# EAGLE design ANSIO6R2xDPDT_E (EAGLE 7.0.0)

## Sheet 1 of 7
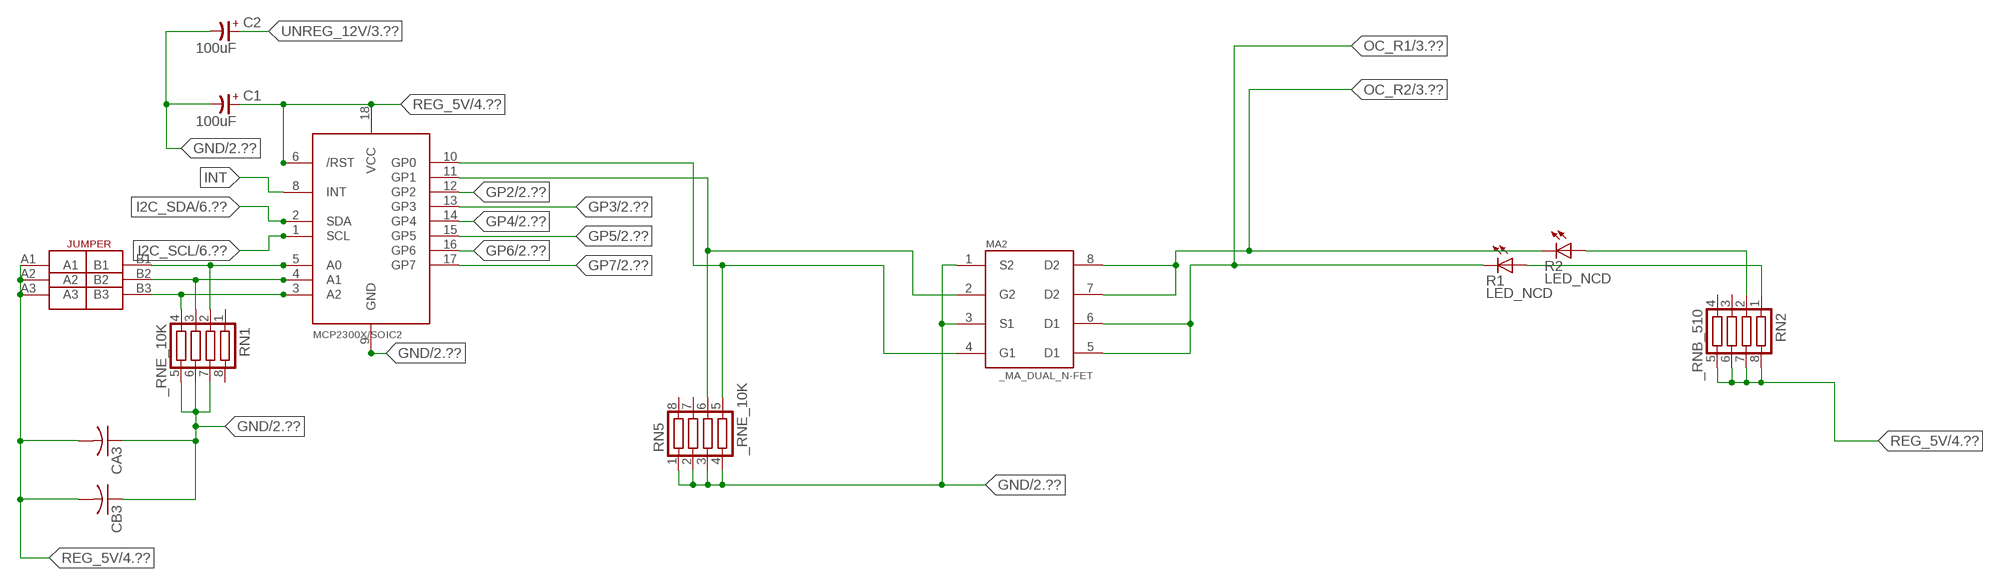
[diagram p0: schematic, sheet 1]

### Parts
C1  100uF  CP-E-025X060  [E-025X060]
C2  100uF  CP-E-025X060  [E-025X060]
CA3  CC1206KRX7R9BB104C1206K  [CC1206KRX7R9BB104]
CB3  TMK316F106ZL-TC1206K  [TMK316F106ZL-T]
IC2  MCP2300X/SO  [SO18W]
MA2  _MA_DUAL_N-FET  [_MA_DUAL_N-FET]
R1  LED_NCD  [CHIPLED_0603]
R2  LED_NCD  [CHIPLED_0603]
RN1  _RNE_10K  [RNE]
RN2  _RNB_510  [RNB]
RN5  _RNE_10K  [RNE]
U$18  JUMPER_3X2  [JUMPER_3X2]

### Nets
GND: C1.- C2.- CA3.1 CB3.1 IC2.9(GND) MA2.1(S2) MA2.3(S1) RN1.5 RN1.6 RN1.7 RN5.1 RN5.2 RN5.3 RN5.4 ; also sheet 2,4,5,6,7
GP2: IC2.12(GP2) ; also sheet 2
GP3: IC2.13(GP3) ; also sheet 2
GP4: IC2.14(GP4) ; also sheet 2
GP5: IC2.15(GP5) ; also sheet 2
GP6: IC2.16(GP6) ; also sheet 2
GP7: IC2.17(GP7) ; also sheet 2
I2C_SCL: IC2.1(SCL) ; also sheet 6,7
I2C_SDA: IC2.2(SDA) ; also sheet 6,7
INT: IC2.8(INT)
N$6: IC2.5(A0) RN1.2 U$18.B1
N$7: IC2.4(A1) RN1.3 U$18.B2
N$8: IC2.3(A2) RN1.4 U$18.B3
N$22: IC2.11(GP1) MA2.2(G2) RN5.6
N$23: IC2.10(GP0) MA2.4(G1) RN5.5
N$31: R2.A RN2.2
N$32: R1.A RN2.1
OC_R1: MA2.5(D1) MA2.6(D1) R1.C ; also sheet 3
OC_R2: MA2.7(D2) MA2.8(D2) R2.C ; also sheet 3
REG_5V: C1.+ CA3.2 CB3.2 IC2.6(/RST) IC2.18(VCC) RN2.5 RN2.6 RN2.7 RN2.8 U$18.A1 U$18.A2 U$18.A3 ; also sheet 4,5,6,7
UNREG_12V: C2.+ ; also sheet 3,4
Unconnected: RN1.1 RN1.8 RN2.3 RN2.4 RN5.7 RN5.8

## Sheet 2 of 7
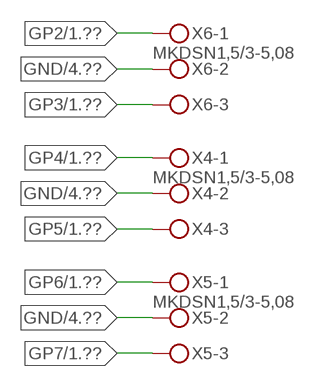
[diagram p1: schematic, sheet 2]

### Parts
X4  MKDSN1,5/3-5,08  [MKDSN1,5/3-5,08]
X5  MKDSN1,5/3-5,08  [MKDSN1,5/3-5,08]
X6  MKDSN1,5/3-5,08  [MKDSN1,5/3-5,08]

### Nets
GND: X4.2 X5.2 X6.2 ; also sheet 1,4,5,6,7
GP2: X6.1 ; also sheet 1
GP3: X6.3 ; also sheet 1
GP4: X4.1 ; also sheet 1
GP5: X4.3 ; also sheet 1
GP6: X5.1 ; also sheet 1
GP7: X5.3 ; also sheet 1

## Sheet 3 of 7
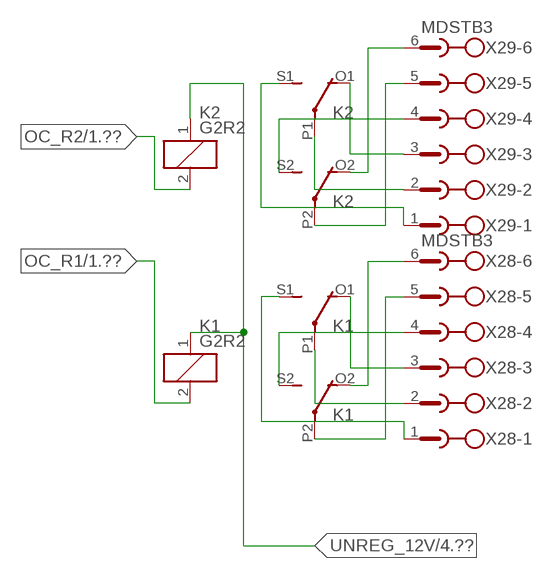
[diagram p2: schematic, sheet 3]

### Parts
K1  G2R2  [G2R2]
K2  G2R2  [G2R2]
X28  MDSTB3  [MDSTB3]
X29  MDSTB3  [MDSTB3]

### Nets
N$203: K1.P2(3:COM) X28.5
N$204: K1.O2(3:NC) X28.6
N$205: K1.S2(3:NO) X28.4
N$206: K1.P1(2:COM) X28.2
N$207: K1.O1(2:NC) X28.3
N$208: K1.S1(2:NO) X28.1
N$209: K2.P2(3:COM) X29.5
N$210: K2.O2(3:NC) X29.6
N$211: K2.S2(3:NO) X29.4
N$212: K2.S1(2:NO) X29.1
N$213: K2.P1(2:COM) X29.2
N$214: K2.O1(2:NC) X29.3
OC_R1: K1.2(1:C2) ; also sheet 1
OC_R2: K2.2(1:C2) ; also sheet 1
UNREG_12V: K1.1(1:C1) K2.1(1:C1) ; also sheet 1,4

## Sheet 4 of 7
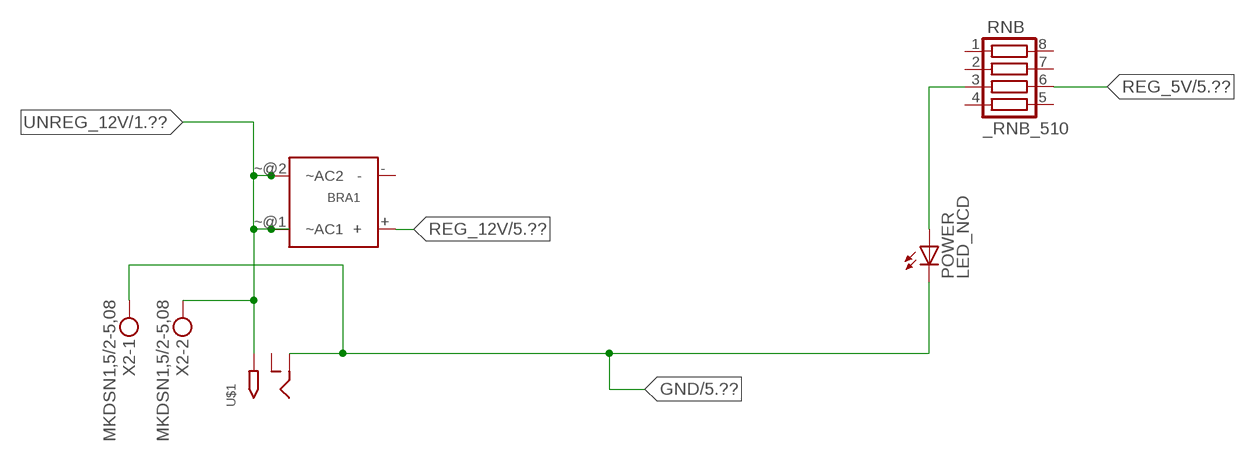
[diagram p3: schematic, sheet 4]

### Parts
BRA1  MB2S_  [MB2S]
POWER  LED_NCD  [CHIPLED_0603]
RNB  _RNB_510  [RNB]
U$1  2.1MMJACK  [PJ-102A]
X2  MKDSN1,5/2-5,08  [MKDSN1,5/2-5,08]

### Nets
GND: POWER.C U$1.RING X2.1 ; also sheet 1,2,5,6,7
N$2: POWER.A RNB.3
REG_5V: RNB.6 ; also sheet 1,5,6,7
REG_12V: BRA1.+ ; also sheet 5
UNREG_12V: BRA1.~@1(~AC1) BRA1.~@2(~AC2) U$1.TIP X2.2 ; also sheet 1,3
Unconnected: BRA1.- RNB.1 RNB.2 RNB.4 RNB.5 RNB.7 RNB.8 U$1.RING_SW

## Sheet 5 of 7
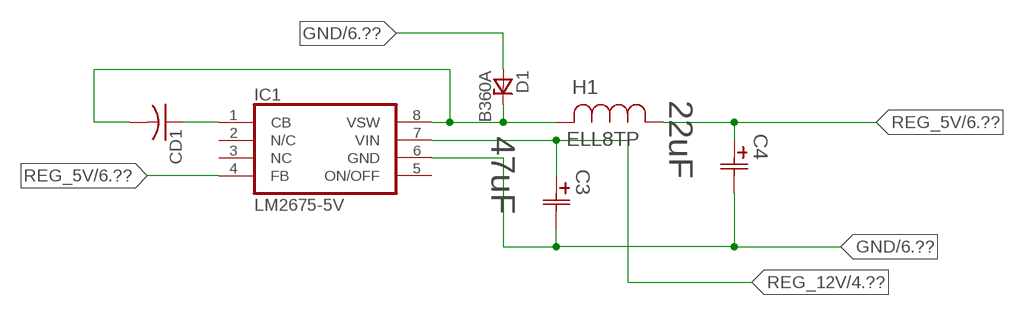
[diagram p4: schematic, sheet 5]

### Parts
C3  47uF  490-5463-6-NDCAP  [C2917(7343)-Y]
C4  22uF  490-5463-6-NDCAP  [C2917(7343)-Y]
CD1  _CD_10NF_50VC1206K  [_CD_10NF_50V]
D1  B360A  [DO214AC_ZENER]
H1  ELL8TP  [IND_ELL8TP]
IC1  LM2675-5V  LM2675  [SO-8]

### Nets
GND: C3.2(C2) C4.2(C2) D1.A IC1.6(GND) ; also sheet 1,2,4,6,7
N$1: CD1.2 D1.C H1.2 IC1.8(VSW)
N$3: CD1.1 IC1.1(CB)
REG_5V: C4.1(C1) H1.1 IC1.4(FB) ; also sheet 1,4,6,7
REG_12V: C3.1(C1) IC1.7(VIN) ; also sheet 4
Unconnected: IC1.2(N/C) IC1.5(ON/OFF)

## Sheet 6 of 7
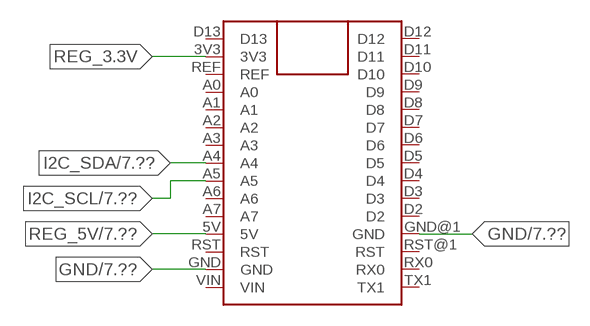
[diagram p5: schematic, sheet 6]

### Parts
FOR_NANO  ARDUINO_NANO  [ARDUINO_NANO]

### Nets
GND: FOR_NANO.GND FOR_NANO.GND@1(GND) ; also sheet 1,2,4,5,7
I2C_SCL: FOR_NANO.A5 ; also sheet 1,7
I2C_SDA: FOR_NANO.A4 ; also sheet 1,7
REG_3.3V: FOR_NANO.3V3
REG_5V: FOR_NANO.5V ; also sheet 1,4,5,7
Unconnected: FOR_NANO.A0 FOR_NANO.A1 FOR_NANO.A2 FOR_NANO.A3 FOR_NANO.A6 FOR_NANO.A7 FOR_NANO.D2 FOR_NANO.D3 FOR_NANO.D4 FOR_NANO.D5 FOR_NANO.D6 FOR_NANO.D7 FOR_NANO.D8 FOR_NANO.D9 FOR_NANO.D10 FOR_NANO.D11 FOR_NANO.D12 FOR_NANO.D13 FOR_NANO.REF FOR_NANO.RST FOR_NANO.RST@1(RST) FOR_NANO.RX0 FOR_NANO.TX1 FOR_NANO.VIN

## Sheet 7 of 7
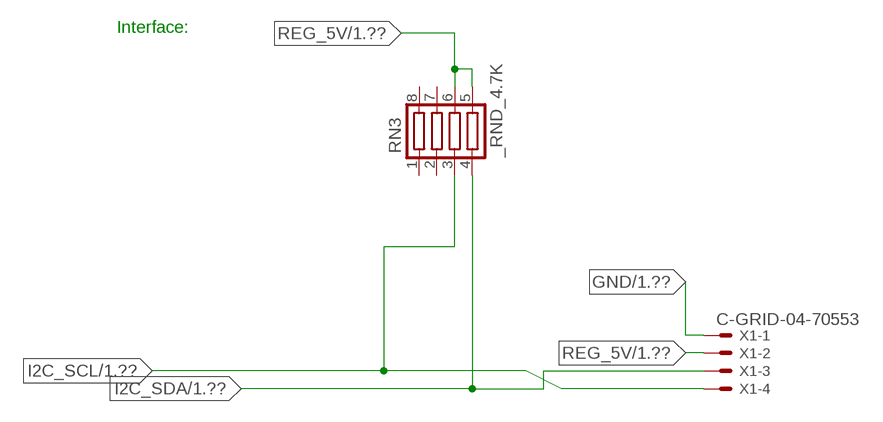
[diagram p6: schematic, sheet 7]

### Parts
RN3  _RND_4.7K  [RND]
X1  C-GRID-04-70553  [70553-04]

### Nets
GND: X1.1 ; also sheet 1,2,4,5,6
I2C_SCL: RN3.3 X1.4 ; also sheet 1,6
I2C_SDA: RN3.4 X1.3 ; also sheet 1,6
REG_5V: RN3.5 RN3.6 X1.2 ; also sheet 1,4,5,6
Unconnected: RN3.1 RN3.2 RN3.7 RN3.8

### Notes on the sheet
- Interface:

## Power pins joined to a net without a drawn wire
NC: IC1.3(NC)

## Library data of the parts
BRA1 = NCD_ULTIMATE_LIBRARY:MB2S: Bridge Rectifier BRA MB2S 200V 500ma Digikey MB2S-TPMSTR-ND/MB2S-TP
C1 C2 = NCD_ULTIMATE_LIBRARY:CP-: Capacitors All Kinds POLARIZED CAP
C3 C4 = NCD_ULTIMATE_bhaskar:490-5463-6-ND: NCD CAP
CA3 = NCD_ULTIMATE_LIBRARY:CC1206KRX7R9BB104: Capacitor CA .1uF 50V SMT C1206K CC1206KRX7R9BB104
CB3 = NCD_ULTIMATE_LIBRARY:TMK316F106ZL-T: Capacitor CB 10uF SMT 1206 TMK316F106ZL-T
CD1 = NCD_ULTIMATE_LIBRARY:_CD_10NF_50V: Capacitor 10nF SMT
D1 = NCD_ULTIMATE_bhaskar:B360A: NCD DIODE B350A/B360A
FOR_NANO = NCD_ULTIMATE_CONNECTORS:ARDUINO_NANO
H1 = NCD_ULTIMATE_bhaskar:ELL8TP: NCD coil
IC1 = NCD_ULTIMATE_bhaskar:LM2675: LM2675 NCD http://www.ti.com/lit/ds/symlink/lm2675.pdf
IC2 = NCD_ULTIMATE_LIBRARY:MCP2300X: Semiconductor Port Expander I/O 8-Bit I2C MCP23008 Inexpensive i2c i/o expander - 8 general purpose i/o pins with optional pullups
K1 K2 = NCD_ULTIMATE_LIBRARY:G2R2: RELAY 2 x switch, Omron
MA2 = NCD_ULTIMATE_LIBRARY:_MA_DUAL_N-FET: FET Dual N-Channel 8-SOIC NMOSFET Digikey 785-1064-2-ND/AO4842
POWER = NCD_ULTIMATE_bhaskar:LED_NCD
R1 R2 = NCD_ULTIMATE_LIBRARY:LED_NCD: LED Digikey 754-1132-2-ND/APT2012SRCPRV
RN1 RN5 = NCD_ULTIMATE_LIBRARY:_RNE_10K: Resistor Array RNE SMT 10K x 4 Single Resistor Source: http://www.ctscorp.com/components/Datasheets/CTSChipArrayDs.pdf Digikey 742C083103JPTR-ND/742C083103JP; OC_FARNELL: unknown; OC_NEWARK: unknown
RN2 RNB = NCD_ULTIMATE_LIBRARY:_RNB_510: Resistor Array RNB SMT 510 x 4 Single Resistor Source: http://www.ctscorp.com/components/Datasheets/CTSChipArrayDs.pdf Digikey 742C083511JPTR-ND/ 742C083511JP; OC_FARNELL: unknown; OC_NEWARK: unknown
RN3 = NCD_ULTIMATE_LIBRARY:_RND_4.7K: Resistor Array RND SMT 4.7K x 4 Single Resistor Source: http://www.ctscorp.com/components/Datasheets/CTSChipArrayDs.pdf Digikey 742C083472JPTR-ND/742C083472JP; OC_FARNELL: unknown; OC_NEWARK: unknown
U$1 = NCD_ULTIMATE_CONNECTORS:2.1MMJACK: 2.1mm x 5.5mm DC jack with internal switch. Digikey part #PJ-102A, 4UCON part #05537 By microbuilder.eu
U$18 = NCD_ULTIMATE_CONNECTORS:JUMPER_3X2
X1 = NCD_ULTIMATE_CONNECTORS:C-GRID-04: CONNECTOR 4-Pos I2C wire to board 2.54 mm (0.100") pitch header Digikey WM1342-ND/0015912045; OC_FARNELL: unknown; OC_NEWARK: unknown
X2 = NCD_ULTIMATE_CONNECTORS:MKDSN1,5/2-5,08: MKDSN 1,5/ 2-5,08 Printklemme
X4-X6 = NCD_ULTIMATE_CONNECTORS:MKDSN1,5/3-5,08: MKDSN 1,5/ 3-5,08 Printklemme Nennstrom: 13,5 A Nennspannung: 250 V Rastermaß: 5,08 mm Polzahl: 3 Anschlussart: Schraubanschluss Montage: Löten Anschlussrichtung Leiter/Platine: 0 ° Artikelnummer: 1729131 Source: http://eshop.phoenixcontact.com .. 1729131.pdf
X28 X29 = NCD_ULTIMATE_LIBRARY:MDSTB3: PHOENIX

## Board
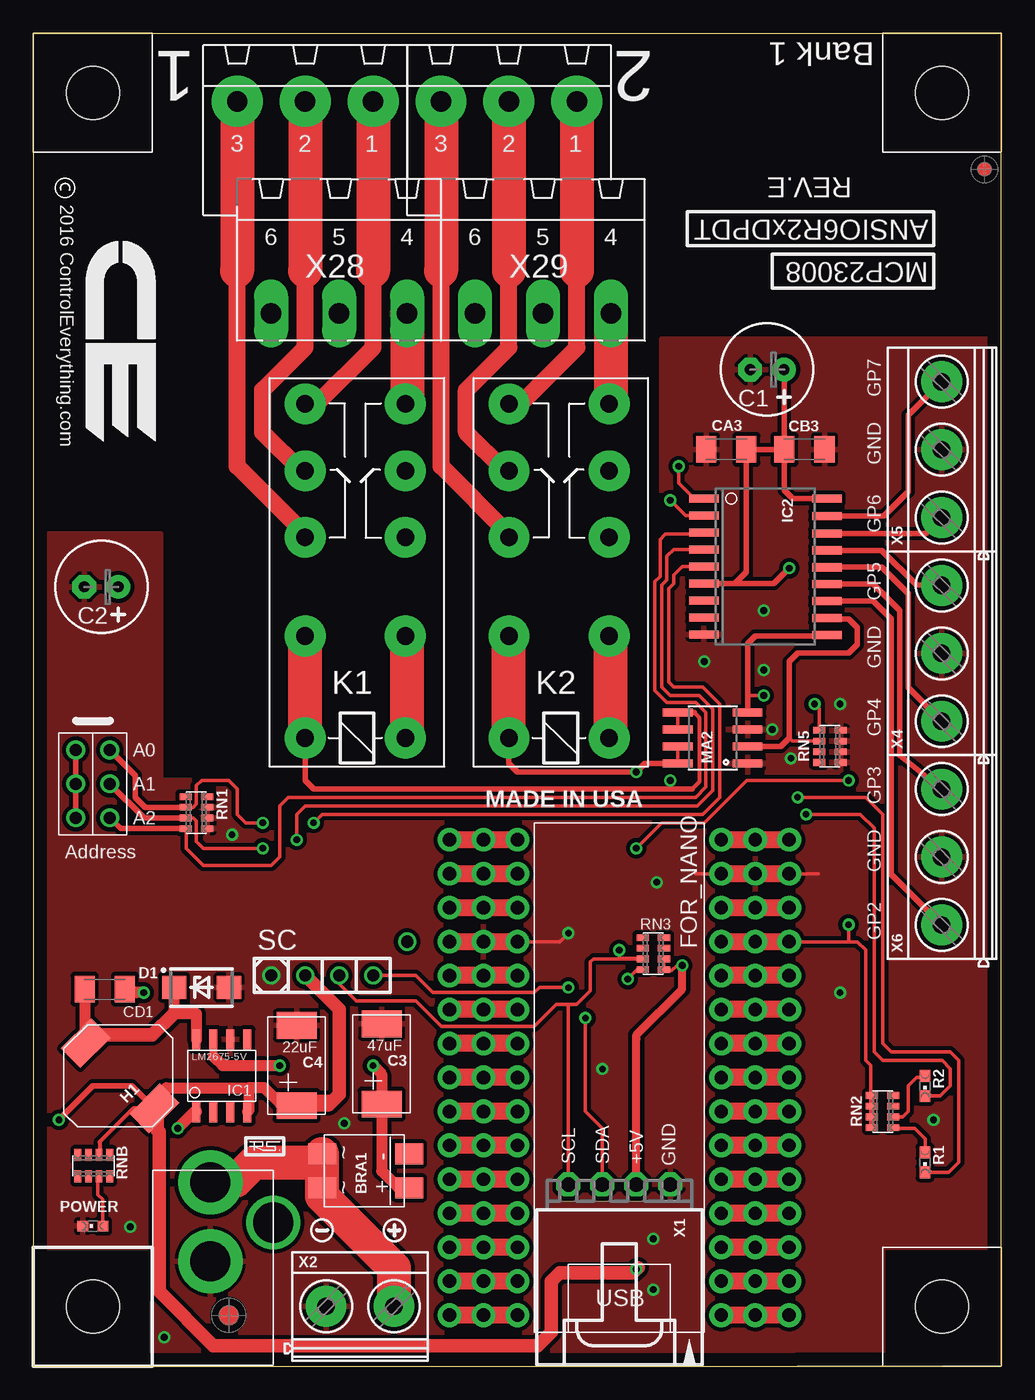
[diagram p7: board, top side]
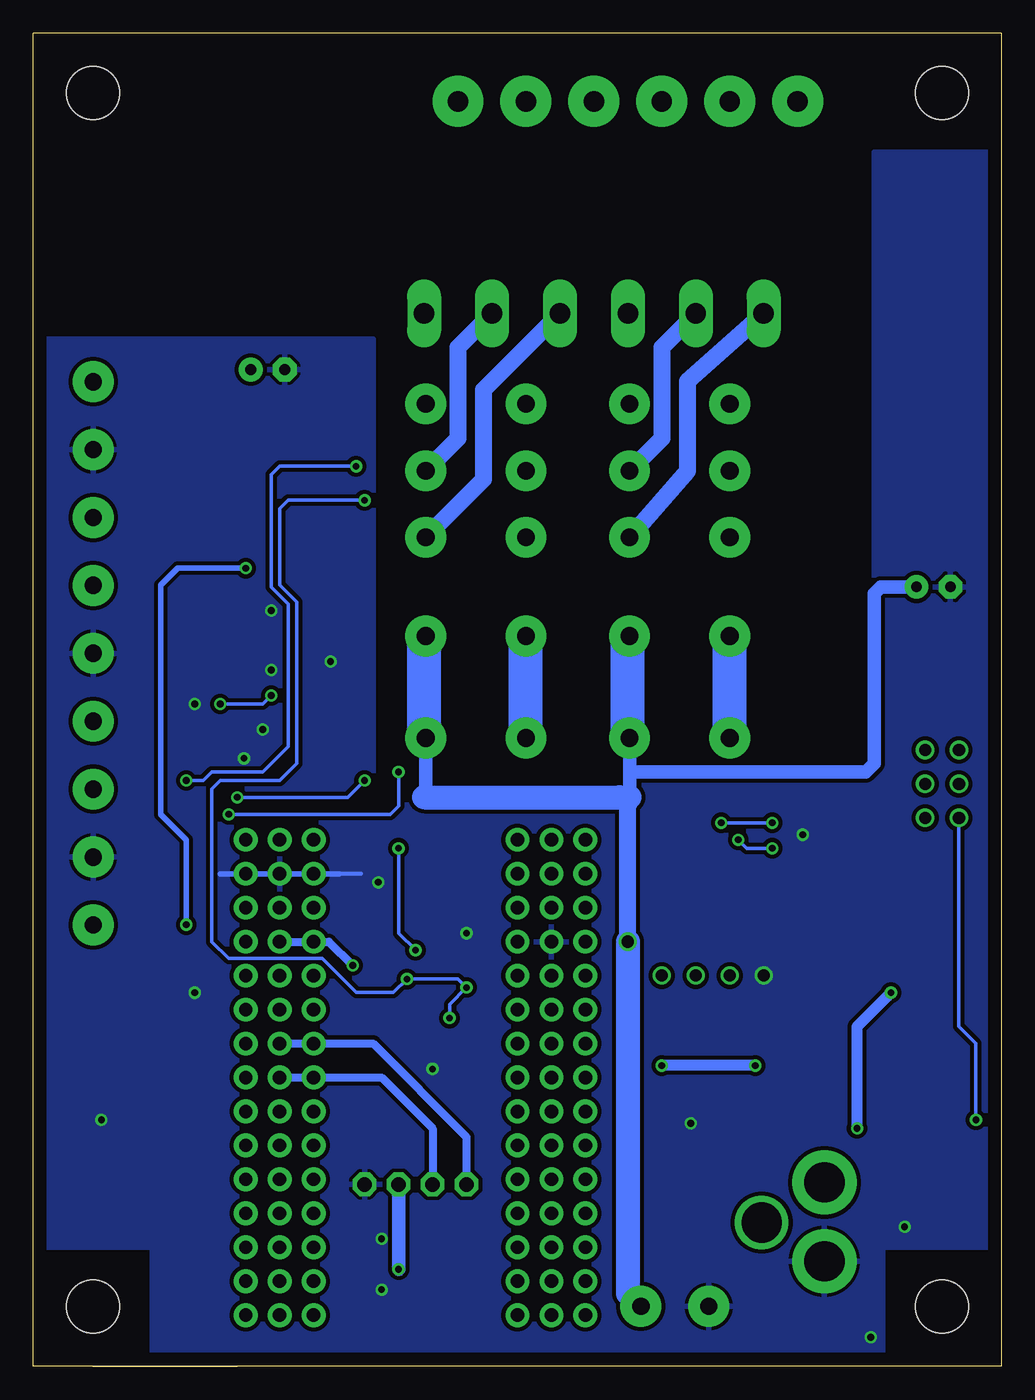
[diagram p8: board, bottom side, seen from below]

Size 72.39 x 99.7 mm. Coordinates in mm from the lower left corner, seen from the top.
Outline: 57.15,0 72.39,0 72.39,99.7 0,99.7 0,85.73 0,0 57.15,0
Outline: 67.94,0 57.15,0
Copper layers (1*16): Top 0.035mm / dielectric 1.5mm / Bottom 0.035mm
Design rules "default": minimum track width 10mil, minimum drill 24mil, track to track 8mil, track to pad 8mil, pad to pad 8mil, via to via 8mil, smd to smd 8mil, copper to edge 40mil, drill to drill 8mil, minimum pad ring 10mil, minimum via ring 8mil, stop-mask expansion 4mil, vias tented up to drill 0mil, thermal gap 10mil
Holes 3.96 mm at 4.45,4.45 4.45,4.45 4.45,4.45 4.45,4.45

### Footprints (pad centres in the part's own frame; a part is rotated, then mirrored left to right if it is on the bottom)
MB2S = smd 1.55 x 2.1: + 0,-6.5; - 2.54,-6.5; ~@1 0,0; ~@2 2.54,0
E-025X060 = drill 0.813 pad 1.778: + -1.27,0 | drill 0.813 pad 1.778 octagon: - 1.27,0
C2917(7343)-Y = smd 2 x 3: 1 -3,0; 2 3,0
CC1206KRX7R9BB104 = smd 1.5 x 2: 1 -1.5,0; 2 1.5,0
TMK316F106ZL-T = smd 1.5 x 2: 1 -1.5,0; 2 1.5,0
_CD_10NF_50V = smd 1.5 x 2: 1 -1.5,0; 2 1.5,0
DO214AC_ZENER = smd 1.8 x 1.7: A 2.05,0; C -2.05,0
ARDUINO_NANO = drill 1 pad 1.778: 3V1 -2.54,-2.54; 3V3 0,-2.54; 5V 0,-27.94; 5V1 -2.54,-27.94; A0 0,-7.62; A1 0,-10.16; A2 0,-12.7; A3 0,-15.24; A4 0,-17.78; A5 0,-20.32; A6 0,-22.86; A7 0,-25.4; A8 -2.54,-7.62; A9 -2.54,-10.16; A10 -2.54,-12.7; A11 -2.54,-15.24; A12 -2.54,-17.78; A13 -2.54,-20.32; A14 -2.54,-22.86; A15 -2.54,-25.4; D1 -2.54,0; D2 20.32,-25.4; D3 20.32,-22.86; D4 20.32,-20.32; D5 20.32,-17.78; D6 20.32,-15.24; D7 20.32,-12.7; D8 20.32,-10.16; D9 20.32,-7.62; D10 20.32,-5.08; D11 20.32,-2.54; D12 20.32,0; D13 0,0; D14 22.86,0; D15 22.86,-2.54; D16 22.86,-5.08; D17 22.86,-7.62; D18 22.86,-10.16; D19 22.86,-12.7; D20 22.86,-15.24; D21 22.86,-17.78; D22 22.86,-20.32; D23 22.86,-22.86; D24 22.86,-25.4; GND 0,-33.02; GND1 -2.54,-33.02; GND@1 20.32,-27.94; GND@2 22.86,-27.94; P$16 2.54,0; P$17 2.54,-2.54; P$18 2.54,-5.08; P$19 2.54,-7.62; P$20 2.54,-10.16; P$21 2.54,-12.7; P$22 2.54,-15.24; P$23 2.54,-17.78; P$24 2.54,-20.32; P$25 2.54,-22.86; P$26 2.54,-25.4; P$27 2.54,-27.94; P$28 2.54,-30.48; P$29 2.54,-33.02; P$30 2.54,-35.56; P$31 17.78,0; P$32 17.78,-2.54; P$33 17.78,-5.08; P$34 17.78,-7.62; P$35 17.78,-10.16; P$36 17.78,-12.7; P$37 17.78,-15.24; P$38 17.78,-17.78; P$39 17.78,-20.32; P$40 17.78,-22.86; P$41 17.78,-25.4; P$42 17.78,-27.94; P$43 17.78,-30.48; P$44 17.78,-33.02; P$45 17.78,-35.56; REF 0,-5.08; REF1 -2.54,-5.08; RST 0,-30.48; RST1 -2.54,-30.48; RST@1 20.32,-30.48; RST@2 22.86,-30.48; RX0 20.32,-33.02; RX1 22.86,-33.02; TX1 20.32,-35.56; TX2 22.86,-35.56; VIN 0,-35.56; VIN1 -2.54,-35.56
IND_ELL8TP = smd 2.054 x 3.2 rotated 45: 1 -2.442,-2.696; 2 2.442,2.442
SO-8 = smd 0.6 x 1.55: 1 -1.905,-2.69; 2 -0.635,-2.69; 3 0.635,-2.69; 4 1.905,-2.69; 5 1.905,2.71; 6 0.635,2.71; 7 -0.635,2.71; 8 -1.905,2.71
SO18W = smd 0.6 x 2.2: 1 -4.445,-4.6; 2 -3.175,-4.6; 3 -1.905,-4.6; 4 -0.635,-4.6; 5 0.635,-4.6; 6 1.905,-4.6; 7 3.175,-4.6; 8 4.445,-4.6; 9 5.715,-4.6; 10 5.775,4.6; 11 4.505,4.6; 12 3.235,4.6; 13 1.965,4.6; 14 0.695,4.6; 15 -0.575,4.6; 16 -1.845,4.6; 17 -3.145,4.6; 18 -4.445,4.6
G2R2 = drill 1.321 pad 3.048: 1 -2.54,-3.683; 2 -2.54,3.81; 3 5.08,-3.683; 4 5.08,3.81; O1 12.471,3.81; O2 12.471,-3.683; P1 17.45,3.81; P2 17.45,-3.683; S1 22.454,3.81; S2 22.454,-3.683
_MA_DUAL_N-FET = smd 0.61 x 2.21: 1 -1.905,-2.616; 2 -0.635,-2.616; 3 0.635,-2.616; 4 1.905,-2.616; 5 1.905,2.616; 6 0.635,2.616; 7 -0.635,2.616; 8 -1.905,2.616
CHIPLED_0603 = smd 0.8 x 0.8: A 0,-0.75; C 0,0.75
CHIPLED_0603' = smd 0.8 x 0.876: A 0,-0.75; C 0,0.75
RNE = smd 0.5 x 0.9: 1 -1.2,-0.8; 2 -0.4,-0.8; 3 0.4,-0.8; 4 1.2,-0.8; 5 1.2,0.8; 6 0.4,0.8; 7 -0.4,0.8; 8 -1.2,0.8
RNB = smd 0.5 x 0.9: 1 -1.2,-0.8; 2 -0.4,-0.8; 3 0.4,-0.8; 4 1.2,-0.8; 5 1.2,0.8; 6 0.4,0.8; 7 -0.4,0.8; 8 -1.2,0.8
RND = smd 0.5 x 0.9: 1 -1.2,-0.8; 2 -0.4,-0.8; 3 0.4,-0.8; 4 1.2,-0.8; 5 1.2,0.8; 6 0.4,0.8; 7 -0.4,0.8; 8 -1.2,0.8
PJ-102A = drill 3 pad 4.8: RING 0.1,-3.39; TIP 0.1,-9.29 | drill 3 pad 3.251: RING_SW -4.6,-6.29
PCB_MOUNTING_HOLE = hole 3.962: 4.445,4.445
JUMPER_3X2 = drill 0.9: A1 0,5.08; A2 0,2.54; A3 0,0; B1 2.54,5.08; B2 2.54,2.54; B3 2.54,0
70553-04 = drill 1.1 pad 1.778 octagon: 1 -3.81,-7.62; 2 -1.27,-7.62; 3 1.27,-7.62; 4 3.81,-7.62
MKDSN1,5/2-5,08 = drill 1.3 pad 3.048: 1 -2.561,0.025; 2 2.519,0.025
MKDSN1,5/3-5,08 = drill 1.3 pad 3.048: 1 -7.641,0.025; 2 -2.561,0.025; 3 2.519,0.025
MDSTB3 = drill 1.524 pad 3.81: 1 -3.81,-10.795; 2 1.27,-10.795; 3 6.35,-10.795 | drill 1.524 pad 2.54 long: 4 -6.35,5.08; 5 -1.27,5.08; 6 3.81,5.08

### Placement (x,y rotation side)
BRA1  21.59,13.34 90 top
C1  54.86,74.55 180 top
C2  5.08,58.29 180 top
C3  26.04,22.61 90 top
C4  19.68,22.48 90 top
CA3  51.82,68.58 0 top
CB3  57.66,68.58 180 top
CD1  5.33,28.19 180 top
D1  12.57,28.32 0 top
FOR_NANO  53.98,3.81 180 top
H1  6.35,21.72 90 top
IC1  14.1,21.72 0 top
IC2  54.74,60.45 270 top
K1  24.13,49.53 90 top
K2  39.37,49.53 90 top
MA2  50.8,46.99 90 top
POWER  4.45,10.48 90 top
R1  LED_NCD  [CHIPLED_0603']  66.67,15.24 180 top
R2  LED_NCD  [CHIPLED_0603']  66.67,20.95 180 top
RN1  12.19,41.4 270 top
RN2  63.5,19.05 90 top
RN3  46.35,30.86 270 top
RN5  59.56,46.35 90 top
RNB  4.51,14.99 0 top
U$1  13.34,4.45 180 top
U$2  [VISION_REF15]  14.61,3.81 0 top
U$3  [ICON_MINUS]  21.59,10.16 180 top
U$4  PCB_MOUNTING_HOLE  [PCB_MOUNTING_HOLE]  72.39,90.81 90 top
U$5  [ICON_PLUS]  26.99,10.16 90 top
U$6  PCB_MOUNTING_HOLE  [PCB_MOUNTING_HOLE]  72.39,0 90 top
U$7  PCB_MOUNTING_HOLE  [PCB_MOUNTING_HOLE]  8.89,90.81 90 top
U$18  3.17,41.02 0 top
U$19  [VISION_REF10]  71.12,89.54 0 top
U$21  [ICON_USA]  33.78,41.78 0 top
X1  43.81,5.97 180 top
X2  24.45,4.45 0 top
X4  67.94,55.88 90 top
X5  67.94,71.12 90 top
X6  67.94,40.64 90 top
X28  21.59,83.82 180 top
X29  36.83,83.82 180 top

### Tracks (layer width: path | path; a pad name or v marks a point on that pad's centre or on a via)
GND  (via drill 0.5, 0.9)
  Top 0.254: 36.2,31.75 39.37,31.75 v40.01,32.38 | FOR_NANO.GND@1 32.38,31.75 | 49.53,36.83 56.52,36.83 58.67,36.83
  Top 1.016: X1.1 47.62,13.74
  Bottom 0.254: 51.44,36.83 FOR_NANO.GND
  Bottom 0.305: 47.88,36.83 49.53,36.83 51.44,36.83
  Bottom 0.406: 49.53,36.83 58.42,36.83
  other vias: 14.86,39.75 54.61,52.07 54.61,56.52 67.31,18.41 50.16,52.7 55.24,47.62 60.33,27.94 56.64,45.47 9.78,2.16 17.78,29.21 46.35,9.53 46.61,36.2 46.35,5.71 42.55,22.23 7.24,10.41 60.33,49.53 23.24,18.16
  pour Bottom (isolate 0.305): -2.54,8.89 8.89,8.89 8.89,0 63.5,0 63.5,8.89 71.75,8.89 71.75,76.84 46.99,76.84 46.99,43.81 9.53,43.81 9.53,90.81 -2.54,90.81
  pour Top (isolate 0.305): -5.08,8.89 8.89,8.89 8.89,0 63.5,0 63.5,8.89 71.75,8.89 71.75,76.84 46.99,76.84 46.99,43.81 9.53,43.81 9.53,62.23 -5.08,62.23
GP2
  Top 0.406: IC2.12 62.8,57.22 64.14,55.88 64.14,36.78 X6.1
GP3
  Top 0.406: IC2.13 62.8,58.49 64.77,56.52 64.77,45.67 X6.3
GP4
  Top 0.406: IC2.14 63.43,59.76 65.41,57.78 65.41,50.75 X4.1
GP5
  Top 0.406: IC2.15 63.43,61.03 66.04,58.42 67.9,58.42 X4.3
GP6
  Top 0.406: IC2.16 66.74,62.3 X5.1
GP7
  Top 0.406: IC2.17 63.6,63.6 65.41,65.41 65.41,71.12 X5.3
I2C_SCL  (via drill 0.5, 0.9)
  Top 0.254: IC2.1 49.4,64.9 48.26,66.04 v48.26,67.31 | 40.01,27.05 40.64,27.05 41.64,28.05 41.64,29.48 41.66,29.5 41.66,30.23 41.89,30.46 RN3.3 45.54,30.48 43.81,30.48 v43.81,31.12 | 40.01,27.05 39.12,27.05 37.47,25.4 30.48,25.4 28.57,27.3 24.13,27.3 22.86,28.58 v22.86,29.21 | X1.4 40.01,27.05 | v60.96,43.81 53.34,43.81 50.16,40.64 46.99,40.64 v45.09,38.73
  Bottom 0.254: v48.26,67.31 53.98,67.31 54.61,66.67 54.61,58.29 53.34,57.02 53.34,46.35 55.24,44.45 59.05,44.45 59.69,43.81 v60.96,43.81 | v45.09,38.73 45.09,32.38 v43.81,31.12
  Bottom 0.61: FOR_NANO.A5 46.99,24.13 40.01,17.14 X1.4
I2C_SDA  (via drill 0.5, 0.9)
  Top 0.254: IC2.2 48.77,63.63 v47.62,64.77 | RN3.4 45.16,29.66 v44.45,28.96 | 40,28.33 v40.01,28.32 37.85,28.32 37.47,27.94 29.84,27.94 28.57,29.21 v25.4,29.21 | X1.3 42.55,17.78 41.27,19.05 v41.27,26.04
  Bottom 0.254: v47.62,64.77 53.34,64.77 53.98,64.14 53.98,58.42 52.7,57.15 52.7,45.09 53.98,43.81 58.42,43.81 59.05,43.18 59.05,31.75 57.78,30.48 50.8,30.48 48.26,27.94 45.47,27.94 v44.45,28.96 40.64,28.96 v40.01,28.32 41.27,27.05 v41.27,26.04
  Bottom 0.61: FOR_NANO.A4 46.35,21.59 42.55,17.78 X1.3
N$1
  Top 0.813: H1.2 3.88,24.77 | D1.C 10.52,26.4 12.19,26.38 IC1.8 | CD1.2 3.83,24.15 4.45,24.77
  Top 1.016: 3.88,24.77 4.45,24.77 8.89,24.77 10.52,26.4
N$2
  Top 0.254: POWER.A 5.2,12.46 4.83,12.83 4.83,14.1 RNB.3
  Top 0.406: 4.95,14.14 RNB.3
N$3  (via drill 0.5)
  Top 0.813: IC1.1 12.04,19.03 v10.79,17.78 | v8.26,27.94 7.72,27.94 CD1.1
  Bottom 0.813: v10.79,17.78 10.79,25.4 v8.26,27.94
N$6  (via drill 0.5)
  Top 0.254: v20.95,40.64 21.59,41.27 50.04,41.27 51.31,42.55 51.31,49.53 50.04,50.8 47.88,50.8 47.5,51.18 47.5,58.17 47.88,58.55 47.88,59.18 48.51,59.82 IC2.5 50.01,59.69 | v17.14,40.64 15.88,40.64 15.24,41.27 15.24,43.18 14.61,43.81 12.57,43.81 12.19,43.43 12.19,42.04 11.94,41.78 11.41,41.78 RN1.2
  Top 0.406: RN1.2 8.36,41.8 7.62,42.55 7.62,44.2 U$18.B1
  Bottom 0.254: v20.95,40.64 v17.14,40.64
N$7  (via drill 0.5)
  Top 0.254: v19.68,39.37 19.68,41.27 20.32,41.91 49.66,41.91 50.8,43.05 50.8,49.15 49.78,50.16 47.62,50.16 46.99,50.8 46.99,58.42 47.37,58.8 47.37,60.58 47.88,61.09 IC2.4 50.01,60.96 | v17.14,38.73 12.7,38.73 12.19,39.24 12.19,40.77 11.94,41.02 11.41,41.02 RN1.3
  Top 0.406: RN1.3 8.27,41 U$18.B2
  Bottom 0.254: v19.68,39.37 19.05,38.73 v17.14,38.73
N$8
  Top 0.254: RN1.4 11.43,40.16 11.43,38.73 12.7,37.47 17.78,37.47 18.41,38.1 18.41,41.91 19.05,42.55 49.53,42.55 50.29,43.31 50.29,48.89 49.53,49.66 47.37,49.66 46.48,50.55 46.48,58.67 46.86,59.05 46.86,61.85 47.24,62.23 50.01,62.23 IC2.3
  Top 0.406: RN1.4 6.53,40.2 U$18.B3
N$22
  Top 0.254: RN5.6 56.75,46.75 56.52,46.99
  Top 0.406: MA2.2 55.88,46.35 56.52,46.99 56.52,52.7 57.15,53.34 60.96,53.34 61.59,53.98 61.59,55.24 60.96,55.88 59.4,55.88 IC2.11
N$23  (via drill 0.5)
  Top 0.254: RN5.5 58.76,49.19 v58.42,49.53 | v54.61,50.16 53.42,50.16
  Top 0.406: MA2.4 53.42,50.16 53.42,54.05 53.98,54.61 59.27,54.61 IC2.10
  Bottom 0.254: v58.42,49.53 55.24,49.53 v54.61,50.16
N$31
  Top 0.254: RN2.2 65,18.65 65.41,19.05 65.41,20.95 66.04,21.59 66.56,21.59 R2.A
N$32
  Top 0.254: R1.A 66.67,17.02 65.91,17.78 64.37,17.78 RN2.1
N$203
  Bottom 1.27: X28.5 25.4,76.2 25.4,69.39 K1.P2
N$204
  Bottom 1.27: X28.6 23.5,73.66 23.5,66.95 K1.O2
N$205
  Top 2.54: X28.4 27.94,72.11 K1.S2
N$206
  Top 1.27: K1.P1 20.02,66.98 17.14,69.85 17.14,73.03 20.32,76.2 20.32,81.92
  Top 2.54: X28.2 20.32,81.92
N$207
  Top 1.27: K1.O1 20.32,62.23 15.24,67.31 15.24,81.92
  Top 2.54: X28.3 15.24,81.92
N$208
  Top 1.27: K1.S1 21.18,71.98 25.4,76.2 25.4,81.92
  Top 2.54: X28.1 25.4,81.92
N$209
  Bottom 1.27: X29.5 40.64,76.2 40.64,69.39 K2.P2
N$210
  Bottom 1.27: X29.6 38.73,73.03 38.73,66.32 K2.O2
N$211
  Top 2.54: X29.4 43.18,72.11 K2.S2
N$212
  Top 1.27: K2.S1 36.2,71.75 40.64,76.2 40.64,81.92
  Top 2.54: X29.1 40.64,81.92
N$213
  Top 1.27: K2.P1 35.26,66.98 32.38,69.85 32.38,73.03 35.56,76.2 35.56,81.92
  Top 2.54: X29.2 35.56,81.92
N$214
  Top 1.27: K2.O1 35.56,62.23 30.48,67.31 30.48,81.92
  Top 2.54: X29.3 30.48,81.92
OC_R1  (via drill 0.5)
  Top 0.254: MA2.5 MA2.6 | R1.C 68.47,14.49 69.22,15.24 69.22,22.86 68.58,23.5 64.14,23.5 63.5,24.13 63.5,41.27 62.23,42.55 v57.15,42.55 | v47.62,43.81 47.62,43.18
  Top 0.305: 49.4,48.89 49.78,48.51 49.78,43.69 49.28,43.18
  Top 0.406: MA2.5 49.4,48.89 | 49.28,43.18 47.62,43.18 20.95,43.18 20.32,43.81 K1.2
  Bottom 0.254: v57.15,42.55 48.9,42.55 v47.62,43.81
OC_R2  (via drill 0.5)
  Top 0.254: MA2.7 MA2.8 | R2.C 67.83,20.2 68.58,20.95 68.58,22.23 67.94,22.86 63.5,22.86 62.87,23.5 62.87,40.26 61.85,41.27 v57.78,41.27
  Top 0.406: MA2.8 45.72,45.09 v45.09,44.45 36.2,44.45 35.56,45.09 K2.2
  Bottom 0.254: v57.78,41.27 45.72,41.27 45.09,41.91 v45.09,44.45
REG_5V  (via drill 0.5, 0.9)
  Top 0.254: RN3.6 RN3.5 47.23,29.59 47.75,29.59 48.13,29.97 v48.51,29.97 | 44.98,24.41 45.09,24.51 | 56.52,31.75 60.96,31.75 | 60.96,31.75 61.59,31.75 62.23,31.12 62.23,22.86 62.61,22.48 62.61,20.34 RN2.5 | v60.96,33.02 60.96,31.75
  Top 0.305: H1.1 7.46,19.27 4.95,16.76 4.95,15.83 RNB.6
  Top 0.406: U$18.A3 U$18.A2 U$18.A1 | RN2.8 RN2.7 RN2.6 RN2.5 | IC2.18 56.77,64.9 56.13,65.53 56.13,68.56 | 56.13,68.56 CB3.2 CA3.2 53.32,59.41 52.45,58.55 IC2.6 55.37,58.55 v56.52,59.69 | C1.+ 56.13,68.56 | v1.91,18.41 4.45,20.95 7.37,20.95 H1.1
  Top 0.61: v48.51,29.97 48.51,28.19 45.09,24.77 45.09,24.51 X1.2
  Top 0.813: 16.13,20.83 9.96,20.83 H1.1 | 16.13,20.83 17.27,20.83 18.41,19.69 20.75,19.69 C4.1 | IC1.4 16.13,19.15 16.13,20.83
  Top 1.016: H1.1 9.27,18.41 9.27,17.65 9.4,17.53 9.4,5.59 13.46,1.52 37.72,1.52 38.73,2.54 38.73,6.35 39.37,6.99 44.83,6.99 v45.09,7.24 45.21,7.37 | 22.05,19.69 22.23,19.69 22.86,20.32 22.86,26.67 v20.32,29.21
  Top 1.27: 20.75,19.69 22.05,19.69
  Bottom 0.254: U$18.A3 3.17,25.4 1.91,24.13 v1.91,18.41
  Bottom 0.406: v56.52,59.69 61.59,59.69 62.87,58.42 62.87,41.27 60.96,39.37 v60.96,33.02
  Bottom 0.61: FOR_NANO.5V 50.29,31.75 v48.51,29.97
  Bottom 1.016: v45.09,7.24 X1.2
REG_12V  (via drill 0.5)
  Top 0.61: IC1.7 13.46,23.16 | 14.1,22.48 14.15,22.48
  Top 0.813: v18.41,22.48 14.15,22.48 13.46,23.16 | v25.4,22.48 26.04,21.84 C3.1 26.04,14.61 27.3,13.34 BRA1.+
  Bottom 0.813: v18.41,22.48 v25.4,22.48
UNREG_12V  (via drill 0.9)
  Top 2.54: X2.2 26.97,7.32 21.59,12.7 BRA1.~@1 21.59,15.24 | 21.59,15.24 BRA1.~@2 | U$1.TIP 15.14,13.87 16.51,15.24 21.59,15.24
  Bottom 0.406: 27.81,42.55 27.81,42.04 27.84,42.06 28.57,42.55
  Bottom 1.016: K1.1 27.81,44.45 | 27.81,44.45 27.81,42.67 27.94,42.55 | K2.1 43.05,42.67 43.18,42.55 | C2.+ 9.02,58.29 9.53,57.78 9.53,45.09 10.16,44.45 27.81,44.45
  Bottom 1.27: v27.94,31.75 27.94,41.96 27.84,42.06
  Bottom 1.778: 43.18,42.55 28.57,42.55 27.94,42.55 27.81,42.55 | v27.94,31.75 27.94,5.44 X2.2

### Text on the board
tNames: Bank 1 | 1 | 2 | REV.E | 2016 ControlEverything.com | ANSIO6R2xDPDT | MCP23008 | GP7 | GND | GP6 | GP5 | GND | GP4 | A0 | A1 | GP3 | A2 | Address | GND | SC | GP2 | SCL | SDA | +5V | GND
